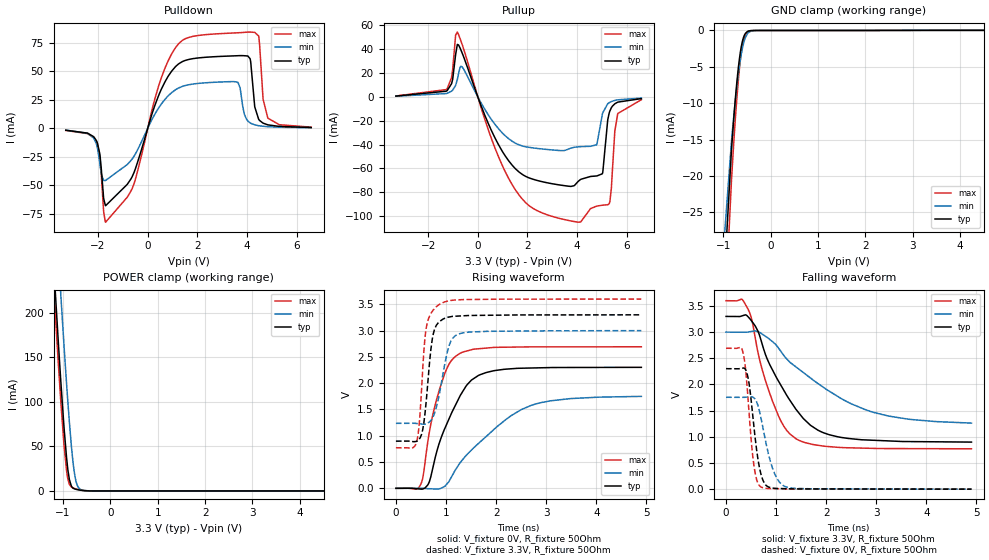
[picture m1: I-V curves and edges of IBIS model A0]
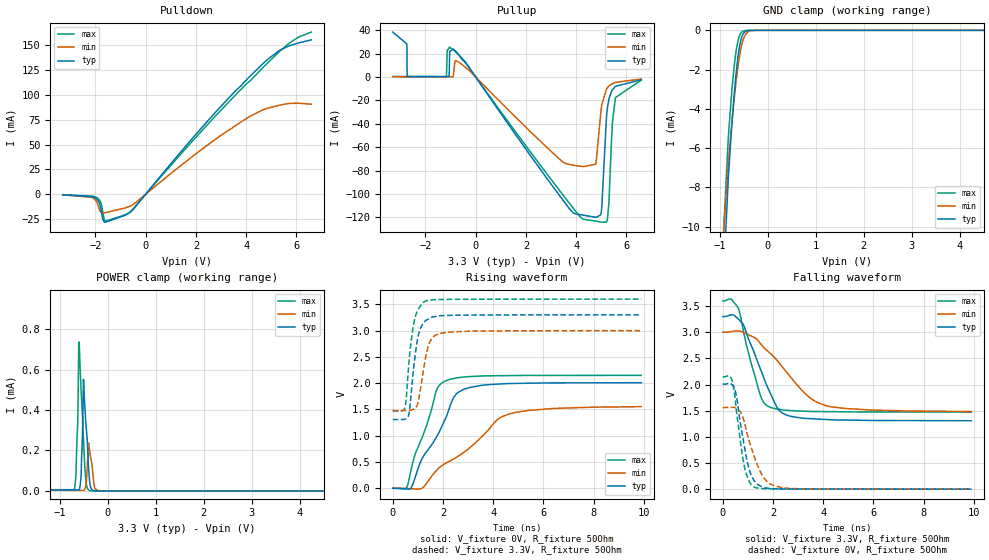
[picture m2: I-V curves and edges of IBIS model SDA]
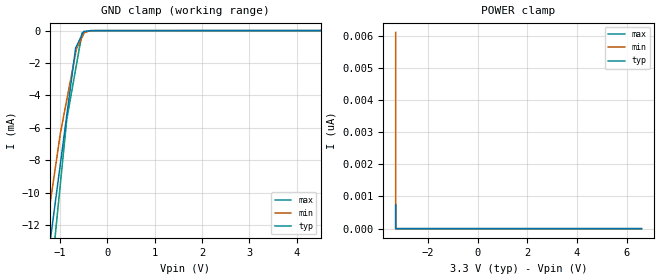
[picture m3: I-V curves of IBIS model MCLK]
|Texas Instruments Incorporated
| Marketing part#   Digital Voltage Range   Package-type   #pins
| TAS5755M   3.0- 3.6V   DFD   56
[IBIS Ver]   4.1
[File name]   tas5755m.ibs
[File Rev]   1.0
[Date]   09/11/2017
[Source]
| Texas Instruments Incorporated.
| 12500 TI Blvd
| Dallas, TX -75243
[Notes]   Revision History:
| Rev 1.0: 09/11/2017
| - Initial version of the model
| - Model generated from simulations in TISPICE
| - C_comp although listed in numerical order of value are
|   obtained from varying PVT conditions. For PVT conditions for
|   each specific value refer the buffer description under
|   respective [Model]. IBIS model user is responsible for using
|   appropriate C_comp to simulate for Signal Integrity.
| - Warnings regarding combined Non-monotonicity of various models have been
|   reviewed and considered minor and can be ignored.
[Disclaimer]
| This model is designed as an aid for customers of Texas Instruments.
| TI and its licensors and suppliers make no warranties, either expressed
| or implied, with respect to this  model, including the warranties of
| merchantability or fitness for a particular purpose. The model is
| provided solely on an "as is" basis. The entire risk as to its quality
| and performance is with the customer.
[Copyright]
 (C) Copyright 2017 Texas Instruments Incorporated. All rights reserved.
|   Device
[Component]   TAS5755M
[Manufacturer]   TI
[Package]  |  56 pin DFD
| variable   typ   min   max
R_pkg   0.1   0.08   0.12
L_pkg   1.0nH   0.8nH   1.2nH
C_pkg   0.2pF   0.16pF   0.24pF
[Pin]  signal_name   model_name   R_pin   L_pin   C_pin
1   PDNZ   RESETZ   NA   NA   NA
2   VR_DIG   NC   NA   NA   NA
3   DVSS_OSC   GND   NA   NA   NA
4   OSC_RES   NC   NA   NA   NA
5   MCLK   MCLK   NA   NA   NA
6   NC   NC   NA   NA   NA
7   NC   NC   NA   NA   NA
8   ADR/FAULT   A0   NA   NA   NA
9   AVDD   POWER   NA   NA   NA
10   VR_ANA   NC   NA   NA   NA
11   FLTP   NC   NA   NA   NA
12   FLTM   NC   NA   NA   NA
13   AVSS   GND   NA   NA   NA
14   AVSS   GND   NA   NA   NA
15   PBTL   SCL   NA   NA   NA
16   SSTIMER   NC   NA   NA   NA
17   BST_A   NC   NA   NA   NA
18   PVDD_AB   POWER   NA   NA   NA
19   PVDD_AB   POWER   NA   NA   NA
20   OUTA   NC   NA   NA   NA
21   OUTA   NC   NA   NA   NA
22   NC   NC   NA   NA   NA
23   PGND   GND   NA   NA   NA
24   PGND   GND   NA   NA   NA
25   PGND   GND   NA   NA   NA
26   OUT_B   NC   NA   NA   NA
27   OUT_B   NC   NA   NA   NA
28   BST_B   NC   NA   NA   NA
29   BST_C   NC   NA   NA   NA
30   OUT_C   NC   NA   NA   NA
31   OUT_C   NC   NA   NA   NA
32   PGND   GND   NA   NA   NA
33   PGND   GND   NA   NA   NA
34   PGND   GND   NA   NA   NA
35   NC   NC   NA   NA   NA
36   OUT_D   NC   NA   NA   NA
37   OUT_D   NC   NA   NA   NA
38   PVDD_CD   POWER   NA   NA   NA
39   PVDD_CD   POWER   NA   NA   NA
40   BST_D   NC   NA   NA   NA
41   GVDD   POWER   NA   NA   NA
42   VREG   NC   NA   NA   NA
43   NC   NC   NA   NA   NA
44   DVSS   GND   NA   NA   NA
45   NC   NC   NA   NA   NA
46   DVSS   GND   NA   NA   NA
47   DVDD   POWER   NA   NA   NA
48   STEST   STEST   NA   NA   NA
49   RESETZ   RESETZ   NA   NA   NA
50   NC   NC   NA   NA   NA
51   NC   NC   NA   NA   NA
52   SCL   SCL   NA   NA   NA
53   SDA   SDA   NA   NA   NA
54   SDIN   SDIN   NA   NA   NA
55   SCLK   MCLK   NA   NA   NA
56   LRCLK   MCLK   NA   NA   NA
| Models and submodels in the file (7): A0 (I/O), SDA (I/O), MCLK (Input), RESETZ (Input), SCL (Input), STEST (Input), SDIN (Input)
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|   Model Selectors
[Model]   A0
Model_type   I/O
Polarity   Non-Inverting
Vinl = 0.8
Vinh = 2.0
Vmeas = 1.65
Vref = 1.65
Cref = 15pF
Rref = 50
|   typ   min   max
C_comp   0.7443p   0.7440p   0.7473p
[Voltage Range]   3.3   3   3.6
[Temperature Range]   27   125   0
[Pullup Reference]   3.3   3   3.6
[Pulldown Reference]   -0   -0   -0
[Power Clamp Reference]   3.3   3   3.6
[GND Clamp Reference]   -0   -0   -0
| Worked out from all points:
|   slope of the pulldown table from 0 to 0.495 V, typ, clamps not added: 15.7 ohm
|   slope of the pullup table from 0 to 0.495 V, typ, clamps not added: 19.2 ohm
|   GND clamp passes 1 mA (typ) near -0.57 V on its own axis
|   POWER clamp passes 1 mA (typ) near -0.65 V on its own axis
|   falling waveform, V_fixture 3.3V, R_fixture 50Ohm: 20-80 % time 811ps typ, 1.47ns min, 522ps max; typ from 3.3 V to 0.899 V
|   rising waveform, V_fixture 0V, R_fixture 50Ohm: 20-80 % time 579ps typ, 1.14ns min, 377ps max; typ from 0 V to 2.3 V
|   rising waveform, V_fixture 3.3V, R_fixture 50Ohm: 20-80 % time 148ps typ, 223ps min, 128ps max; typ from 0.897 V to 3.3 V
|   falling waveform, V_fixture 0V, R_fixture 50Ohm: 20-80 % time 174ps typ, 260ps min, 141ps max; typ from 2.3 V to 0 V
[Pulldown]
|   Voltage   I(typ)   I(min)   I(max)
-3.3V     -1.623mA   -1.525mA   -1.817mA
-2.062V   -10.94mA   -13.92mA   -12.15mA
-1.696V   -67.79mA   -45.62mA   -82.24mA
-627mV    -42.42mA   -26.84mA   -52.87mA
422.4mV   27.81mA    17.28mA    35.85mA
1.155V    54.84mA    34.3mA     71.78mA
3.61V     63.69mA    40.63mA    83.79mA
4.036V    63.43mA    6.497mA    84.39mA
4.471V    8.001mA    2.345mA    80.95mA
4.65V     4.591mA    1.839mA    25.59mA
4.848V    3.066mA    1.48mA     8.894mA
6.59V     752.9uA    535.7uA    1.094mA
[GND Clamp]
|   Voltage   I(typ)   I(min)   I(max)
-3.3V     -1.551A    -1.405A    -1.594A
-1.171V   -56mA      -45.46mA   -66.77mA
-825mV    -16.3mA    -15.14mA   -20.45mA
-775.5mV  -11.9mA    -11.65mA   -15.17mA
-726mV    -8.044mA   -8.507mA   -10.47mA
-686.4mV  -5.443mA   -6.289mA   -7.237mA
-646.8mV  -3.36mA    -4.389mA   -4.571mA
-607.2mV  -1.849mA   -2.851mA   -2.569mA
-567.6mV  -895.5uA   -1.703mA   -1.257mA
-478.5mV  -126uA     -388.1uA   -168.9uA
-270.6mV  -19.24uA   -14.79uA   -27.02uA
6.59V     0A         0A         0A
[Pullup]
|   Voltage   I(typ)   I(min)   I(max)
-3.3V     660.5uA    526.6uA    750.8uA
-1.251V   5.021mA    2.888mA    6.511mA
-1.013V   14.72mA    5.612mA    22.97mA
-825mV    43.95mA    14.51mA    54.28mA
-636.9mV  37.04mA    25.19mA    44.25mA
1.492V    -59.72mA   -38.56mA   -77.2mA
4.036V    -71.05mA   -41.88mA   -105mA
4.788V    -66.29mA   -40.2mA    -91.58mA
5.016V    -64.51mA   -14.91mA   -90.81mA
5.293V    -13.68mA   -4.886mA   -89.46mA
5.64V     -4.42mA    -2.489mA   -13.99mA
6.59V     -1.469mA   -1.032mA   -2.37mA
[POWER Clamp]
|   Voltage   I(typ)   I(min)   I(max)
-3.3V     2.297A     2.39A      2.274A
-1.231V   284.3mA    385mA      259.4mA
-1.102V   170.1mA    269.1mA    146.1mA
-1.043V   120.6mA    217.4mA    97.79mA
-973.5mV  68.05mA    159.3mA    48.46mA
-924mV    36.97mA    120.1mA    22.39mA
-894.3mV  22.65mA    97.82mA    12.6mA
-825mV    5.667mA    51.79mA    4.439mA
-755.7mV  2.306mA    19.3mA     2.723mA
-666.6mV  1.123mA    3.318mA    1.463mA
-468.6mV  69.68uA    162.8uA    92.65uA
6.59V     0A         0A         0A
[Ramp]
R_load = 50
|   typ   min   max
dV/dt_r   1.3808/5.76205e-10   1.04936/1.14252e-09   1.61519/3.76139e-10
dV/dt_f   1.44054/8.09573e-10   1.0428/1.46744e-09   1.69758/5.21429e-10
[Falling Waveform]
V_fixture = 3.3V
V_fixture_min = 3V
V_fixture_max = 3.6V
R_fixture = 50Ohm
C_fixture = 0F
|   Time   V(typ)   V(min)   V(max)
0s        3.3V       3V         3.6V
311.2ps   3.308V     2.998V     3.631V
435.7ps   3.296V     3.001V     3.445V
639.2ps   3.015V     3.008V     2.606V
923.9ps   2.284V     2.82V      1.691V
1.151ns   1.892V     2.557V     1.206V
1.395ns   1.527V     2.336V     964mV
1.951ns   1.075V     1.941V     821.5mV
2.902ns   935.8mV    1.479V     779.9mV
4.9ns     899.1mV    1.262V     770.7mV
[Rising Waveform]
V_fixture = 0V
V_fixture_min = 0V
V_fixture_max = 0V
R_fixture = 50Ohm
C_fixture = 0F
|   Time   V(typ)   V(min)   V(max)
0s        867pV      40.83nV    646.3pV
495.3ps   -14.66mV   1.072mV    73.14mV
555ps     -4.913mV   -1.96mV    303mV
667.9ps   125.4mV    -7.82mV    1.071V
863.5ps   853.9mV    -8.887mV   1.861V
1.053ns   1.305V     121.5mV    2.349V
1.274ns   1.746V     477.4mV    2.564V
1.685ns   2.163V     885mV      2.658V
2.702ns   2.289V     1.578V     2.69V
4.9ns     2.301V     1.749V     2.692V
[Rising Waveform]
V_fixture = 3.3V
V_fixture_min = 3V
V_fixture_max = 3.6V
R_fixture = 50Ohm
C_fixture = 0F
|   Time   V(typ)   V(min)   V(max)
0s        897.3mV    1.236V     770.4mV
403.4ps   891.6mV    1.234V     853.6mV
455.6ps   925.7mV    1.229V     1.126V
511.8ps   1.026V     1.223V     1.879V
621.3ps   1.836V     1.233V     3.129V
725.3ps   2.835V     1.329V     3.365V
875ps     3.175V     1.834V     3.503V
1.058ns   3.258V     2.702V     3.568V
1.252ns   3.277V     2.936V     3.586V
4.9ns     3.3V       2.999V     3.6V
[Falling Waveform]
|Gnd
V_fixture = 0V
V_fixture_min = 0V
V_fixture_max = 0V
R_fixture = 50Ohm
C_fixture = 0F
|   Time   V(typ)   V(min)   V(max)
0s        2.302V     1.755V     2.692V
332.4ps   2.312V     1.754V     2.632V
387.3ps   2.288V     1.756V     2.316V
447.5ps   2.088V     1.762V     1.615V
555ps     1.209V     1.745V     462.7mV
621.3ps   676.6mV    1.639V     151.1mV
702.3ps   269.9mV    1.334V     39.33mV
926.2ps   21.43mV    403.1mV    10.6mV
1.204ns   8.623mV    40.95mV    4.629mV
4.9ns     53.1uV     297.3uV    13.79uV
[Model]   SDA
Model_type   I/O
Polarity   Non-Inverting
Vinl = 0.8
Vinh = 2.0
Vmeas = 1.65
Vref = 1.65
Cref = 15pF
Rref = 50
|   typ   min   max
C_comp   0.7443p   0.7440p   0.7473p
[Voltage Range]   3.3   3   3.6
[Temperature Range]   27   125   0
[Pullup Reference]   3.3   3   3.6
[Pulldown Reference]   -0   -0   -0
[Power Clamp Reference]   3.3   3   3.6
[GND Clamp Reference]   -0   -0   -0
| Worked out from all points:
|   slope of the pulldown table from 0 to 0.495 V, typ, clamps not added: 32.5 ohm
|   slope of the pullup table from 0 to 0.495 V, typ, clamps not added: 31.9 ohm
|   GND clamp passes 1 mA (typ) near -0.60 V on its own axis
|   POWER clamp passes 1 mA (typ) near -3.29 V on its own axis
|   falling waveform, V_fixture 3.3V, R_fixture 50Ohm: 20-80 % time 1.01ns typ, 1.72ns min, 668ps max; typ from 3.3 V to 1.31 V
|   rising waveform, V_fixture 0V, R_fixture 50Ohm: 20-80 % time 1.29ns typ, 2.35ns min, 888ps max; typ from 0 V to 2.01 V
|   rising waveform, V_fixture 3.3V, R_fixture 50Ohm: 20-80 % time 299ps typ, 342ps min, 283ps max; typ from 1.31 V to 3.3 V
|   falling waveform, V_fixture 0V, R_fixture 50Ohm: 20-80 % time 440ps typ, 642ps min, 368ps max; typ from 2.01 V to 0 V
[Pulldown]
|   Voltage   I(typ)   I(min)   I(max)
-3.3V     -559.9uA   -542.7uA   -469.7uA
-2.122V   -2.468mA   -3.204mA   -1.888mA
-1.983V   -3.945mA   -6.17mA    -2.853mA
-1.785V   -14.05mA   -17.97mA   -8.449mA
-1.706V   -24.93mA   -18.84mA   -17.74mA
-1.637V   -28.06mA   -18.67mA   -26.01mA
-686.4mV  -19.39mA   -12.65mA   -19.01mA
2.363V    70.7mA     47.61mA    67.34mA
4.155V    118.7mA    78.38mA    114mA
5.333V    144.8mA    89.61mA    143.7mA
6.095V    152.3mA    91.5mA     158.2mA
6.59V     155.2mA    90.54mA    163.1mA
[GND Clamp]
|   Voltage   I(typ)   I(min)   I(max)
-3.3V     -1.514A    -1.357A    -1.56A
-1.607V   -47.21mA   -35.03mA   -43.52mA
-825mV    -7.581mA   -6.783mA   -5.501mA
-745.8mV  -4.664mA   -4.596mA   -2.961mA
-706.2mV  -3.403mA   -3.61mA    -1.948mA
-666.6mV  -2.316mA   -2.718mA   -1.15mA
-627mV    -1.437mA   -1.937mA   -591.7uA
-587.4mV  -790.1uA   -1.288mA   -259.8uA
-508.2mV  -156.3uA   -434.6uA   -32.58uA
-409.2mV  -10.58uA   -65.64uA   -1.24uA
-270.6mV  -46.46nA   -2.385uA   0A
6.59V     0A         0A         0A
[Pullup]
|   Voltage   I(typ)   I(min)   I(max)
-3.3V     38.34mA    165.8uA    389.7uA
-2.736V   28.28mA    154uA      344uA
-2.726V   348.7uA    153.8uA    343.5uA
-1.162V   326.1uA    144.3uA    317.2uA
-1.063V   357.5uA    144.2uA    24.35mA
-894.3mV  23.79mA    154.1uA    23.32mA
4.026V    -117.4mA   -75.91mA   -116mA
4.778V    -119.9mA   -74.6mA    -123.2mA
4.976V    -117.8mA   -30.66mA   -124mA
5.224V    -29.62mA   -9.709mA   -123.2mA
5.561V    -8.046mA   -4.65mA    -17.58mA
6.59V     -2.35mA    -1.735mA   -2.682mA
[POWER Clamp]
|   Voltage   I(typ)   I(min)   I(max)
-3.3V     1.038mA    9.254mA    692.2uA
-2.874V   479.6uA    1.182mA    323.7uA
-2.627V   255.8uA    434.3uA    140.4uA
-2.023V   7.025uA    93.11uA    6.497uA
-696.3mV  4.878uA    2.32uA     6.22uA
-627mV    4.868uA    2.316uA    346.2uA
-597.3mV  4.824uA    2.315uA    736.5uA
-557.7mV  72.19uA    2.312uA    496.7uA
-508.2mV  551.7uA    2.308uA    257.9uA
-389.4mV  71.88uA    217.3uA    3.215uA
-211.2mV  69.71nA    2.032uA    0A
6.59V     0A         0A         0A
[Ramp]
R_load = 50
|   typ   min   max
dV/dt_r   1.20505/1.28979e-09   0.932073/2.35176e-09   1.28889/8.87513e-10
dV/dt_f   1.1951/1.01652e-09   0.909529/1.72053e-09   1.27543/6.67234e-10
[Falling Waveform]
V_fixture = 3.3V
V_fixture_min = 3V
V_fixture_max = 3.6V
R_fixture = 50Ohm
C_fixture = 0F
|   Time   V(typ)   V(min)   V(max)
0s        3.3V       3V         3.6V
332.3ps   3.331V     3.012V     3.634V
631.3ps   3.247V     3.024V     3.448V
830.9ps   3.138V     2.994V     3.012V
1.472ns   2.334V     2.803V     1.834V
1.851ns   1.881V     2.614V     1.574V
2.371ns   1.456V     2.339V     1.517V
3.451ns   1.349V     1.755V     1.487V
4.086ns   1.332V     1.601V     1.483V
9.9ns     1.308V     1.484V     1.474V
[Rising Waveform]
V_fixture = 0V
V_fixture_min = 0V
V_fixture_max = 0V
R_fixture = 50Ohm
C_fixture = 0F
|   Time   V(typ)   V(min)   V(max)
0s        951pV      57.66nV    -337.4nV
565.5ps   -13.03mV   -3.808mV   23.65mV
730.3ps   4.516mV    -8.506mV   343.5mV
1.146ns   541.2mV    -6.853mV   936.5mV
1.742ns   976.2mV    337.4mV    1.863V
2.078ns   1.301V     466.5mV    2.037V
2.371ns   1.673V     543.9mV    2.083V
2.615ns   1.828V     613.4mV    2.105V
4.634ns   1.992V     1.413V     2.144V
9.9ns     2.008V     1.553V     2.148V
[Rising Waveform]
V_fixture = 3.3V
V_fixture_min = 3V
V_fixture_max = 3.6V
R_fixture = 50Ohm
C_fixture = 0F
|   Time   V(typ)   V(min)   V(max)
0s        1.308V     1.479V     1.474V
467.9ps   1.312V     1.478V     1.512V
541.1ps   1.326V     1.477V     1.722V
622.6ps   1.374V     1.48V      2.249V
816.5ps   2.216V     1.502V     3.08V
984.4ps   2.827V     1.593V     3.372V
1.318ns   3.193V     2.506V     3.564V
1.541ns   3.25V      2.838V     3.583V
2.058ns   3.286V     2.96V      3.593V
9.9ns     3.3V       3V         3.6V
[Falling Waveform]
|Gnd
V_fixture = 0V
V_fixture_min = 0V
V_fixture_max = 0V
R_fixture = 50Ohm
C_fixture = 0F
|   Time   V(typ)   V(min)   V(max)
0s        2.009V     1.56V      2.148V
325.6ps   2.014V     1.564V     2.132V
475.2ps   1.918V     1.56V      1.812V
715ps     1.228V     1.467V     874.5mV
849.4ps   850.4mV    1.304V     465.1mV
1.047ns   395.2mV    934.3mV    155.2mV
1.256ns   160.8mV    625.9mV    37.79mV
1.755ns   20.76mV    150.1mV    8.108mV
2.528ns   3.802mV    17.6mV     2.766mV
9.9ns     21.89uV    142.1uV    -337.4nV
[Model]   MCLK
Model_type   Input
Vinl = .8
Vinh = 2
|   typ   min   max
C_comp   0.7443p   0.7440p   0.7473p
[Voltage Range]   3.3   3   3.6
[Temperature Range]   27   125   0
[Power Clamp Reference]   3.3   3   3.6
[GND Clamp Reference]   -0   -0   -0
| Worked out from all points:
|   GND clamp passes 1 mA (typ) near -0.65 V on its own axis
[GND Clamp]
|   Voltage   I(typ)   I(min)   I(max)
-3.3V     -1.514A    -1.357A    -1.56A
-1.441V   -19.09mA   -15.41mA   -22.82mA
-1.238V   -13.78mA   -11.35mA   -16.83mA
-988.3mV  -8.243mA   -6.357mA   -9.481mA
-852.9mV  -5.236mA   -4.277mA   -5.487mA
-665.8mV  -1.08mA    -1.402mA   -2.396mA
-649.3mV  -979.8uA   -1.149mA   -2.125mA
-529.9mV  -249.7uA   -419.5uA   -152.6uA
-497.8mV  -53.24uA   -223uA     -123.4uA
-358.6mV  -12.14uA   -10.45uA   -5.776uA
-237.4mV  -3.461uA   -2.36uA    -4.816uA
6.6V      0A         0A         0A
[POWER Clamp]
|   Voltage   I(typ)   I(min)   I(max)
-3.3V     728.6pA    6.099nA    754.7pA
-3.3V     0A         0A         0A
-3.3V     0A         0A         0A
6.6V      0A         0A         0A
